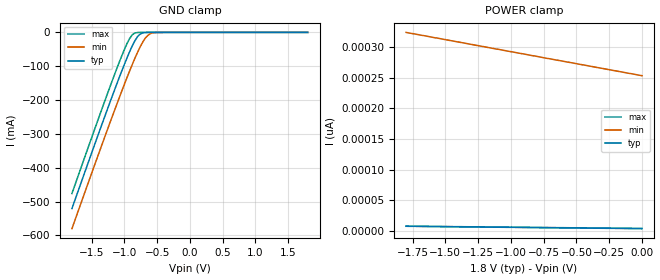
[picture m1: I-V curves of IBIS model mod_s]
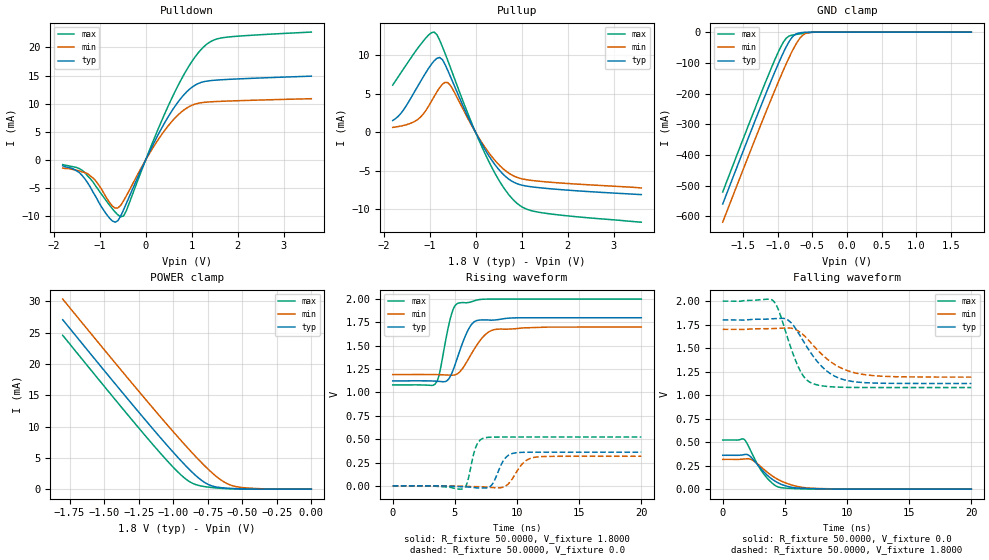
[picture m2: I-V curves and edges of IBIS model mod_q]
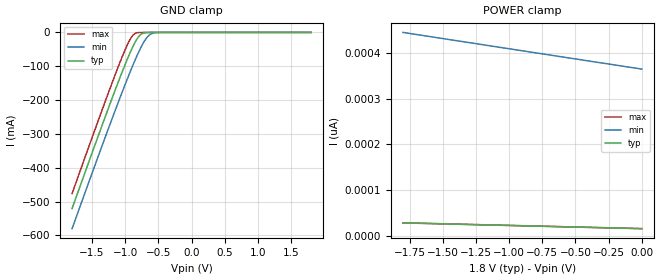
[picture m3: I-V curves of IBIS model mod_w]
| IBIS (I/O, Buffer, Information, Specification) Model, officially
| electronic behavioral standard for Buffer structures of digital pins.
[IBIS ver]  4.0
[File name] m95xxx_g10_tssop8.ibs
[File Rev]  1.0
[Date]   08 Jun 2015
[Source]   CAD & Design Services (Catania) - STMicroelectronics
[Notes]
   (Note1)  This IBIS model includes the TSSOP8 ceramic package parasitic data
   (Note2)  This IBIS model considers: VCC=1.80(TYP), 1.70(MIN), 2.00(MAX)
   (Note3)  This IBIS model has some Notes about the non-monotonicity
   of the I-V curves, but they are not indicative of problems
   inside the model;
[Copyright] (c) 2015 STMicroelectronics
|   Component M95XXX
[Component] M95XXX
[Manufacturer] STMicroelectronics
[Package]
| variable   typ   min   max
R_pkg   0.0   0.0   0.0
L_pkg   0.0H   0.0H   0.0H
C_pkg   0.0F   0.0F   0.0F
[Pin]   signal_name   model_name   R_pin   L_pin   C_pin
1   SN   mod_s   NA   NA   NA
2   Q   mod_q   NA   NA   NA
3   WN   mod_w   NA   NA   NA
4   GND   GND   NA   NA   NA
5   D   mod_s   NA   NA   NA
6   C   mod_s   NA   NA   NA
7   HOLDN   mod_h   NA   NA   NA
8   VCC   POWER   NA   NA   NA
[Package Model]  182696_TSSOP8
[Define Package Model]  182696_TSSOP8
[Manufacturer]  STMicroelectronics
[OEM]  STMicroelectronics
[Description]  8 pin TSSOP package
[Number Of Pins]  8
[Pin Numbers]
|Pin Num   Terminal Name
1   | net1
2   | net2
3   | net3
4   | net4_GND
5   | net5
6   | net6
7   | net7
8   | net8_VDD
[Model Data]
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[End Model Data]
[End Package Model]
| Models and submodels in the file (4): mod_s (Input), mod_q (I/O), mod_w (Input), mod_h (Input)
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|   Model mod_s
[Model]   mod_s
Model_type Input
Vinl   =   0.540V
Vinh   =   1.260V
C_comp   2.120pF   2.024pF   2.323pF
[Temperature Range]  25.0000   0.1050k   -40.0000
[Voltage Range]   1.8000V   1.7000V   2.0000V
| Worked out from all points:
|   GND clamp passes 1 mA (typ) near -0.70 V on its own axis
[GND_clamp]
|Voltage   I(typ)   I(min)   I(max)
-1.8V     -520.5mA   -579.9mA   -476.1mA
-1.24V    -217.2mA   -277.5mA   -171.5mA
-1.08V    -134.2mA   -194.1mA   -89.03mA
-960mV    -75.37mA   -133.6mA   -33.28mA
-880mV    -40.08mA   -95.18mA   -7.121mA
-800mV    -12.85mA   -59.37mA   -321.2uA
-760mV    -5.046mA   -43.15mA   -53.02uA
-720mV    -1.515mA   -28.7mA    -8.596uA
-640mV    -95.71uA   -8.329mA   -224.5nA
-560mV    -5.562uA   -1.25mA    -5.861nA
-480mV    -321.5nA   -139.5uA   -153.9pA
1.8V      3.691pA    257.4pA    3.633pA
[POWER_clamp]
|Voltage   I(typ)   I(min)   I(max)
-1.8V     7.58pA     324.2pA    7.783pA
-700mV    5.176pA    280.9pA    5.483pA
-680mV    5.133pA    280.2pA    5.442pA
0V        3.691pA    253.5pA    4.042pA
|   Model mod_q
[Model]   mod_q
Model_type I/O
Enable   Active-Low
Vinl   =   0.540V
Vinh   =   1.260V
Vmeas  =   0.900V
Cref   =   30pF
C_comp   3.063pF   2.793pF   3.358pF
[Temperature Range]   25.0000   0.1050k   -40.0000
[Voltage Range]   1.8000V   1.7000V   2.0000V
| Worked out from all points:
|   slope of the pulldown table from 0 to 0.27 V, typ, clamps not added: 60.4 ohm
|   slope of the pullup table from 0 to 0.27 V, typ, clamps not added: 94.3 ohm
|   GND clamp passes 1 mA (typ) near -0.63 V on its own axis
|   POWER clamp passes 1 mA (typ) near -0.77 V on its own axis
|   rising waveform, R_fixture 50.0000, V_fixture 1.8000: 20-80 % time 1.14ns typ, 1.49ns min, 829ps max; typ from 1.12 V to 1.8 V
|   rising waveform, R_fixture 50.0000, V_fixture 0.0: 20-80 % time 765ps typ, 1.01ns min, 564ps max; typ from 0 V to 0.36 V
|   falling waveform, R_fixture 50.0000, V_fixture 0.0: 20-80 % time 1.76ns typ, 2.18ns min, 1.44ns max; typ from 0.36 V to 0 V
|   falling waveform, R_fixture 50.0000, V_fixture 1.8000: 20-80 % time 2.28ns typ, 2.65ns min, 1.49ns max; typ from 1.8 V to 1.12 V
[Pulldown]
|Voltage   I(typ)   I(min)   I(max)
-1.8V     -1mA       -1.4mA     -800uA
-1.44V    -2.2mA     -1.9mA     -1.5mA
-1.26V    -4mA       -2.4mA     -2.8mA
-720mV    -10.8mA    -8.157mA   -8.643mA
-600mV    -10.73mA   -8.475mA   -9.721mA
-480mV    -8.845mA   -7.247mA   -9.928mA
120mV     2.051mA    1.662mA    2.482mA
540mV     8.336mA    6.572mA    10.47mA
900mV     12.18mA    9.28mA     16.13mA
1.26V     13.91mA    10.24mA    20.09mA
1.74V     14.3mA     10.47mA    21.79mA
3.6V      14.9mA     10.9mA     22.72mA
[Pullup]
|Voltage   I(typ)   I(min)   I(max)
-1.8V     1.541mA    650uA      6.136mA
-1.32V    5.333mA    1.436mA    10.39mA
-1.02V    8.318mA    3.405mA    12.63mA
-900mV    9.282mA    4.649mA    13.01mA
-780mV    9.719mA    5.807mA    11.95mA
-660mV    8.778mA    6.498mA    10.2mA
-540mV    7.154mA    6.04mA     8.309mA
240mV     -2.578mA   -2.242mA   -3.193mA
600mV     -5.437mA   -4.728mA   -7.081mA
900mV     -6.653mA   -5.831mA   -9.201mA
1.44V     -7.21mA    -6.37mA    -10.42mA
3.6V      -8.07mA    -7.21mA    -11.65mA
[GND_clamp]
|Voltage   I(typ)   I(min)   I(max)
-1.8V     -560mA     -619.1mA   -520.9mA
-1.24V    -237mA     -297.3mA   -196.5mA
-1.08V    -148.5mA   -208.5mA   -108.4mA
-960mV    -85.65mA   -144.1mA   -48.54mA
-880mV    -47.76mA   -103.1mA   -19.64mA
-800mV    -18.02mA   -64.94mA   -10.12mA
-760mV    -9.035mA   -47.59mA   -8.516mA
-720mV    -4.395mA   -32.1mA    -7.15mA
-640mV    -1.177mA   -9.975mA   -4.574mA
-560mV    -260.9uA   -1.867mA   -2.212mA
-440mV    -32.49uA   -185.8uA   -105.6uA
1.8V      141.6pA    90.63nA    112.5pA
[POWER_clamp]
|Voltage   I(typ)   I(min)   I(max)
-1.8V     27.04mA    30.34mA    24.55mA
-1.38V    15.74mA    19.07mA    13.22mA
-1.14V    9.437mA    12.77mA    6.935mA
-980mV    5.408mA    8.678mA    3.048mA
-880mV    3.078mA    6.217mA    1.172mA
-800mV    1.495mA    4.345mA    516.6uA
-740mV    688.2uA    3.042mA    311.5uA
-660mV    257.8uA    1.558mA    143.9uA
-580mV    116.9uA    614.2uA    50.95uA
-500mV    45.75uA    257.8uA    12.5uA
-360mV    2.111uA    62.1uA     99.91nA
0V        141.6pA    1.297nA    151.7pA
[Ramp]
| variable   typ   min   max
dV/dt_r   0.2164/0.8782n   0.1919/1.1568n   0.3134/0.6367n
dV/dt_f   0.4057/2.4641n   0.2970/2.9439n   0.5524/1.7521n
R_load = 50.0000
[Rising Waveform]
R_fixture= 50.0000
V_fixture= 1.8000   | new T=105 (min)
V_fixture_min= 1.7000
V_fixture_max= 2.0000
|time   V(typ)   V(min)   V(max)
0s        1.124V     1.192V     1.081V
3.4ns     1.122V     1.191V     1.088V
3.76ns    1.118V     1.19V      1.203V
4.48ns    1.141V     1.186V     1.704V
4.88ns    1.248V     1.186V     1.894V
5.28ns    1.401V     1.207V     1.956V
6.4ns     1.738V     1.429V     1.974V
7.36ns    1.777V     1.608V     1.999V
8.08ns    1.775V     1.67V      2V
20ns      1.8V       1.7V       2V
[Rising Waveform]
R_fixture= 50.0000
V_fixture= 0.0
V_fixture_min= 0.0   |  New T=105 (min)
V_fixture_max= 0.0
|time   V(typ)   V(min)   V(max)
0s        5.912nV    194.5nV    5.854nV
5.56ns    -9.308mV   -4.644mV   -35.45mV
5.98ns    -11.42mV   -6.423mV   28.01mV
6.74ns    -21.59mV   -8.602mV   432.4mV
7.5ns     -22.62mV   -12.58mV   516.6mV
8.06ns    27.07mV    -18.71mV   521.9mV
8.9ns     269.1mV    -13.15mV   522.7mV
9.7ns     348.9mV    91.43mV    522.8mV
11.54ns   360.3mV    308.4mV    522.8mV
20ns      360.5mV    316.9mV    522.8mV
[Falling Waveform]
R_fixture= 50.0000
V_fixture= 0.0   | New T =105 (min)
V_fixture_min= 0.0
V_fixture_max= 0.0
|time   V(typ)   V(min)   V(max)
0s        360.5mV    316.9mV    522.8mV
1.72ns    367.4mV    320.7mV    529.9mV
2.2ns     350.2mV    320.6mV    422.6mV
2.8ns     260.9mV    269.3mV    263.3mV
3.28ns    188.2mV    214.4mV    165.5mV
4.04ns    100.2mV    135.9mV    57.14mV
4.6ns     57.82mV    93.13mV    18.65mV
5.88ns    13.76mV    32.85mV    5.534mV
7.28ns    5.246mV    9.388mV    1.282mV
20ns      127.1nV    1.699uV    4.73nV
[Falling Waveform]
R_fixture= 50.0000
V_fixture= 1.8000   | New T = 105 (min)
V_fixture_min= 1.7000
V_fixture_max= 2.0000
|time   V(typ)   V(min)   V(max)
0s        1.8V       1.7V       2V
4.04ns    1.813V     1.708V     2.007V
4.48ns    1.816V     1.711V     1.909V
5.24ns    1.799V     1.714V     1.602V
6.2ns     1.637V     1.671V     1.268V
6.68ns    1.533V     1.617V     1.172V
7.3ns     1.41V      1.527V     1.121V
9ns       1.202V     1.327V     1.087V
11.02ns   1.137V     1.227V     1.082V
20ns      1.124V     1.192V     1.081V
|   Model mod_w
[Model]   mod_w
Model_type Input
Vinl   =   0.540V
Vinh   =   1.260V
C_comp   2.120pF   2.024pF   2.323pF
[Temperature Range]  25.0000   0.1050k   -40.0000
[Voltage Range]   1.8000V   1.7000V   2.0000V
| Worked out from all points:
|   GND clamp passes 1 mA (typ) near -0.70 V on its own axis
[GND_clamp]
|Voltage   I(typ)   I(min)   I(max)
-1.8V     -520.9mA   -580.3mA   -476.5mA
-1.2V     -196.3mA   -256.7mA   -150.7mA
-1.04V    -114.2mA   -173.8mA   -69.64mA
-960mV    -75.5mA    -133.8mA   -33.44mA
-880mV    -40.19mA   -95.27mA   -7.262mA
-800mV    -12.93mA   -59.44mA   -437.7uA
-760mV    -5.115mA   -43.21mA   -157.1uA
-720mV    -1.572mA   -28.76mA   -100.4uA
-640mV    -131.4uA   -8.363mA   -67.87uA
-560mV    -23uA      -1.269mA   -44.38uA
-480mV    -5.764uA   -149uA     -22.96uA
1.8V      15.18pA    369.3pA    13.84pA
[POWER_clamp]
|Voltage   I(typ)   I(min)   I(max)
-1.8V     27.74pA    445.2pA    28.05pA
-1.36V    24.65pA    425.4pA    24.91pA
-1.34V    24.5pA     424.6pA    24.77pA
0V        15.18pA    364.8pA    15.26pA
